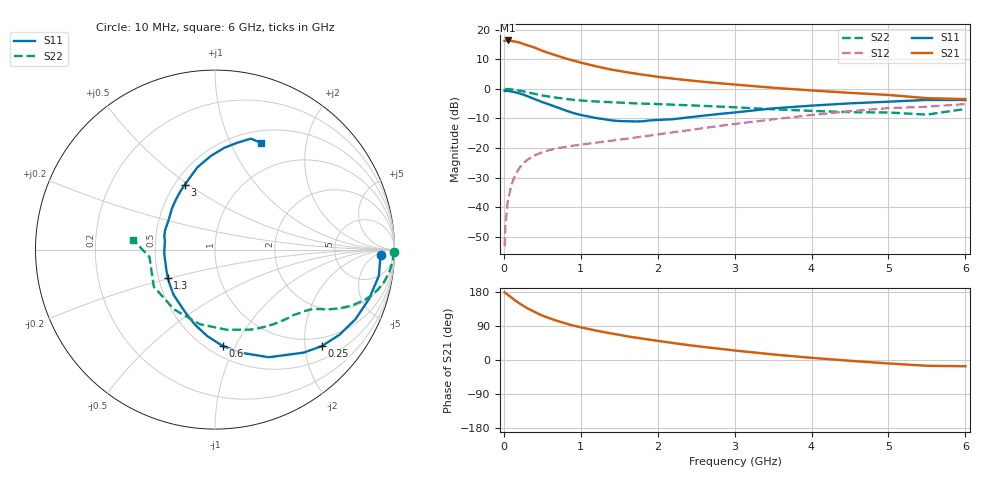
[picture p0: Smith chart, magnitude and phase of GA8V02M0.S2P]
! Infineon Technologies  Discrete & RF Semiconductors
! BF775
! Si NPN RF Bipolar Junction Transistor in SOT23
! VCE = 8 V  IC = 2 mA
! Common Emitter S-Parameters:  May  1996
# GHz  S  MA  R  50
!  f  S11  S21  S12  S22
! GHz  MAG  ANG  MAG  ANG  MAG  ANG  MAG  ANG
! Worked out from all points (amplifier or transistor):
!   36 points, 10 MHz to 6 GHz, reference 50 ohm
!   highest |S21| = 16.4 dB at 50 MHz (marker M1)
!   |S21| within 3 dB of that: start of sweep to 455.4 MHz
!   unconditionally stable (mu >= 1): 1.208 GHz to 3.259 GHz
!   at 250 MHz: K = 0.28, MSG = 20.2 dB, |S12| = -25.3 dB
!   at 1.4 GHz: K = 1.08, MAG = 10.3 dB, |S12| = -17.5 dB
!   at 6 GHz: K = 0.94, MSG = 0.8 dB, |S12| = -5.1 dB
!   S11 on the Smith chart (normalised r, x): 10 MHz: 22, -9; 250 MHz: 0.79, -2.37; 600 MHz: 0.59, -0.89; 1.3 GHz: 0.56, -0.20; 3 GHz: 0.56, +0.48; 6 GHz: 0.64, +1.31
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0.01  0.9264 -1.8  6.467 178.6  0.0022 92.3  0.9981 -0.7
0.02  0.9219 -3.5  6.444 176.7  0.0048 86.2  0.9936 -1.4
0.05  0.9246 -9.1  6.571 172.2  0.0124 85.8  0.9924 -3.7
0.1  0.9011 -17.8  6.429 164.8  0.0242 80.1  0.9792 -7.3
0.15  0.8733 -26.4  6.272 156.6  0.0353 74.0  0.9601 -10.7
0.2  0.8402 -34.4  6.088 149.8  0.0455 70.5  0.9354 -13.7
0.25  0.8021 -42.1  5.754 143.4  0.0545 66.5  0.9075 -16.4
0.3  0.7578 -49.2  5.474 137.1  0.0627 63.3  0.8797 -18.6
0.4  0.6707 -63.4  4.985 126.8  0.0751 57.7  0.823 -22.3
0.5  0.5978 -74.7  4.4 117.2  0.0849 53.7  0.7729 -24.9
0.6  0.5389 -85.4  3.966 109.7  0.0929 50.9  0.7366 -26.7
0.8  0.4328 -104.9  3.273 96.7  0.1047 47.9  0.6777 -29.3
0.9  0.3918 -114.1  3.012 91.0  0.1098 47.5  0.6538 -30.4
1.1  0.3416 -132.4  2.579 81.9  0.1188 47.4  0.6233 -32.6
1.3  0.3076 -148.7  2.248 73.7  0.1287 47.5  0.6026 -34.8
1.7  0.2815 177.5  1.823 59.5  0.15 50.1  0.5687 -39.9
2.2  0.3067 147.2  1.488 44.8  0.1843 51.4  0.5404 -48.0
3  0.399 114.9  1.184 25.1  0.2551 49.8  0.4884 -65.9
3.5  0.4686 102.1  1.044 14.7  0.3056 46.3  0.452 -81.4
4.5  0.5688 84.9  0.856 -2.1  0.4202 35.0  0.4037 -124.4
5.5  0.6498 72.1  0.696 -15.3  0.4988 18.4  0.3673 -173.7
6  0.6473 66.6  0.671 -16.5  0.5532 13.8  0.4571 173.5
